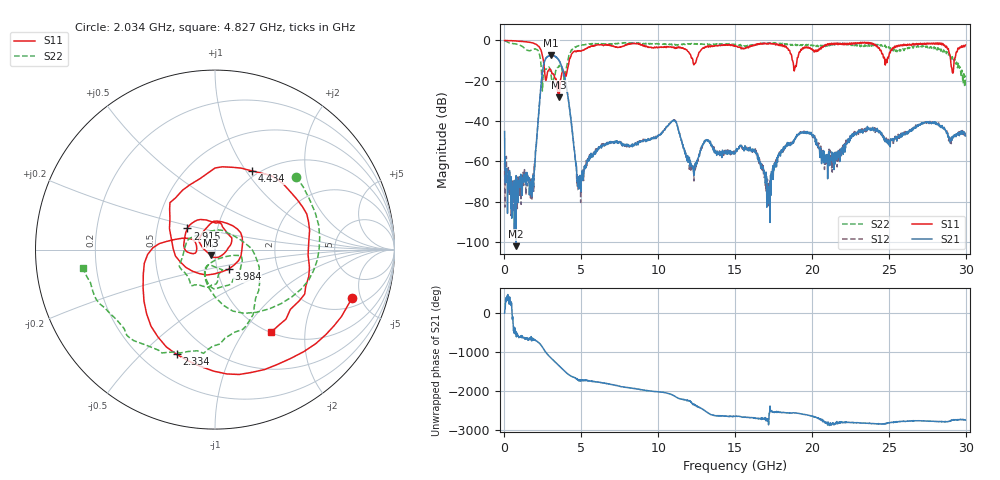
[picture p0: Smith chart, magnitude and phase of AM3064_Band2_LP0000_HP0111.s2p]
# Hz S DB R 50.0
!freq dBS11 angS11 dBS21 angS21 dBS12 angS12 dBS22 angS22
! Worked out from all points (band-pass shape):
!   1600 points, 10 MHz to 29.98 GHz, reference 50 ohm
!   highest |S21| = -7.41 dB at 3.046 GHz (marker M1); lowest = -102.0 dB at 741 MHz (marker M2)
!   |S21| within 3 dB of the highest: 2.608 GHz to 3.585 GHz (976.6 MHz wide, 31.5 % of centre)
!   lowest |S11| = -28.1 dB at 3.553 GHz (marker M3), VSWR 1.08, Z = 47.5 - j2.91 ohm
!   |S11| at or under -10 dB: 2.538 GHz to 4.215 GHz (1.677 GHz wide, 49.7 % of centre); 18.74 GHz to 19.02 GHz (283.5 MHz wide, 1.5 % of centre); 29.02 GHz to 29.25 GHz (228 MHz wide, 0.783 % of centre)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
!   |S22| runs from -25.1 to -0.2 dB; largest |S21 - S12| = 0.0096
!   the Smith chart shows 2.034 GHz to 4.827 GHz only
!   S11 on the Smith chart (normalised r, x): 2.034 GHz: 2.65, -4.18; 2.334 GHz: 0.34, -0.64; 2.915 GHz: 0.72, +0.18; 3.984 GHz: 1.13, -0.25; 4.434 GHz: 0.93, +1.07; 4.827 GHz: 1.02, -1.35
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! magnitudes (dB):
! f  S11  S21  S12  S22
! 10 MHz  0.0  -45.1  -60.7  -0.2
! 741 MHz  -0.3  -102.0  -81.6  -1.8
! 1.772 GHz  -1.2  -77.4  -71.0  -4.8
! 2.034 GHz  -1.8  -54.0  -54.7  -4.3
! 2.334 GHz  -4.1  -26.1  -26.0  -9.0
! 2.915 GHz  -14.3  -7.7  -7.7  -13.4
! 3.046 GHz  -15.3  -7.4  -7.4  -18.2
! 3.553 GHz  -28.1  -10.0  -9.9  -12.5
! 3.984 GHz  -17.5  -20.8  -20.8  -16.2
! 4.434 GHz  -6.3  -46.2  -46.9  -4.2
! 4.827 GHz  -5.1  -67.5  -74.4  -2.6
! 5.015 GHz  -5.2  -69.8  -69.6  -2.4
! 10 GHz  -3.4  -47.2  -47.0  -1.7
! 11.09 GHz  -3.9  -39.7  -39.5  -1.9
! 12.27 GHz  -10.8  -63.7  -62.1  -1.6
! 15 GHz  -2.5  -56.0  -54.8  -1.9
! 16.28 GHz  -2.3  -54.7  -54.4  -2.2
! 17.18 GHz  -1.8  -72.5  -76.1  -1.6
! 19.99 GHz  -4.2  -46.9  -46.8  -2.2
! 21.12 GHz  -1.8  -58.8  -53.9  -2.7
! 25 GHz  -7.9  -50.2  -50.9  -3.1
! 29.98 GHz  -2.3  -47.3  -46.5  -17.4
